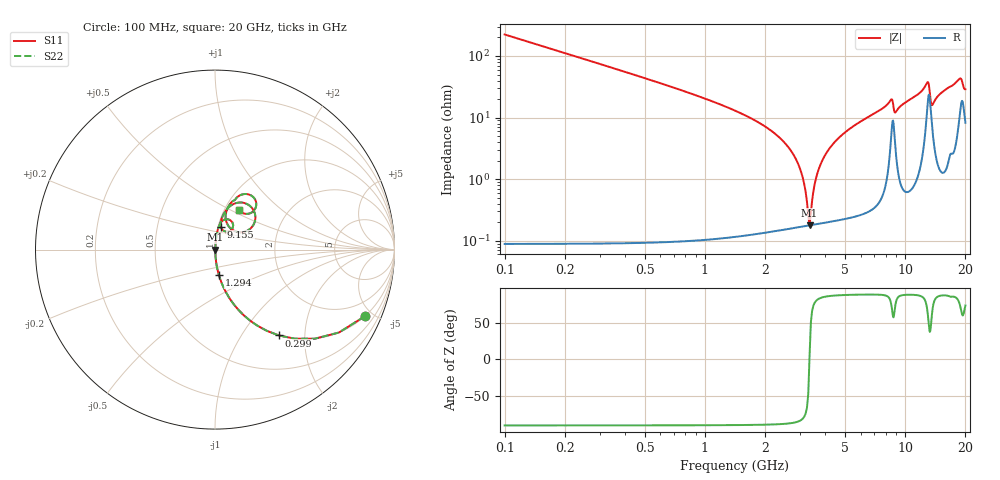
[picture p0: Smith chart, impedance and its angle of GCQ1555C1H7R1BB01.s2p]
!Murata Part Number: GCQ1555C1H7R1BB01
!These Parameters are Measured in Series Mode Connection
!Data Generated on Jan 08, 2026
!  o--ll--o
!Port1  Port2
!  o------o
!Operation Temp=25[degC], DC Bias Voltage=0[V]
!Freq. Start=100[MHz] Stop=20[GHz] 401[Steps]
# Hz S RI R 50
!Freq.(Hz) S11(Real) S11(Imag) S21(Real) S21(Imag) S12(Real) S12(Imag) S22(Real) S22(Imag)
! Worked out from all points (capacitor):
!   401 points, 100 MHz to 20 GHz, reference 50 ohm
!   read as one part in series: C = 7.1 pF near 199.5 MHz
!   lowest |Z| = 178 mohm at 3.334 GHz (marker M1)
!   series resonance near 3.33 GHz, so ESL is about 320 pH
!   S11 on the Smith chart (normalised r, x): 100 MHz: 1.00, -4.48; 299 MHz: 1.00, -1.49; 1.294 GHz: 1.00, -0.29; 9.155 GHz: 1.03, +0.27; 20 GHz: 1.16, +0.55
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1e8  0.8337 -0.3722  0.1663 0.3722  0.1663 0.3722  0.8337 -0.3722
2.99e8  0.3562 -0.4783  0.6438 0.4783  0.6438 0.4783  0.3562 -0.4783
5.975e8  0.1171 -0.3202  0.8829 0.3202  0.8829 0.3202  0.1171 -0.3202
1.294e9  0.0222 -0.1436  0.9778 0.1436  0.9778 0.1436  0.0222 -0.1436
2.73675e9  0.00229 -0.0265  0.9977 0.0265  0.9977 0.0265  0.00229 -0.0265
3.03525e9  0.00184 -0.0125  0.9982 0.0125  0.9982 0.0125  0.00184 -0.0125
3.33375e9  0.00177 0.000157  0.9982 -0.000157  0.9982 -0.000157  0.00177 0.000157
3.43325e9  0.00182 0.00412  0.9982 -0.00412  0.9982 -0.00412  0.00182 0.00412
3.5825e9  0.00194 0.00986  0.9981 -0.00986  0.9981 -0.00986  0.00194 0.00986
3.73175e9  0.00212 0.0154  0.9979 -0.0154  0.9979 -0.0154  0.00212 0.0154
4.279e9  0.00322 0.0342  0.9968 -0.0342  0.9968 -0.0342  0.00322 0.0342
6.7665e9  0.0147 0.107  0.9853 -0.107  0.9853 -0.107  0.0147 0.107
8.50775e9  0.0748 0.1682  0.9252 -0.1682  0.9252 -0.1682  0.0748 0.1682
8.856e9  0.0585 0.1006  0.9415 -0.1006  0.9415 -0.1006  0.0585 0.1006
9.1545e9  0.0319 0.1276  0.9681 -0.1276  0.9681 -0.1276  0.0319 0.1276
1.005e10  0.0359 0.1693  0.9641 -0.1693  0.9641 -0.1693  0.0359 0.1693
1.288575e10  0.193 0.2449  0.807 -0.2449  0.807 -0.2449  0.193 0.2449
1.338325e10  0.143 0.0963  0.857 -0.0963  0.857 -0.0963  0.143 0.0963
1.3632e10  0.0838 0.1211  0.9162 -0.1211  0.9162 -0.1211  0.0838 0.1211
1.67165e10  0.108 0.2748  0.892 -0.2748  0.892 -0.2748  0.108 0.2748
1.875625e10  0.2117 0.294  0.7883 -0.294  0.7883 -0.294  0.2117 0.294
2e10  0.1328 0.2216  0.8672 -0.2216  0.8672 -0.2216  0.1328 0.2216
